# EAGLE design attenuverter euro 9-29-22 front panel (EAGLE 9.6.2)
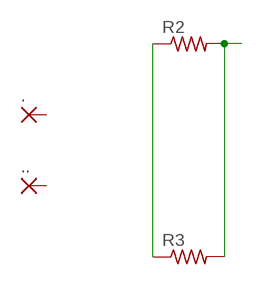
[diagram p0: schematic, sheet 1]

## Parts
.  WIREPADSMD1,27-254  [SMD1,27-2,54]
..  WIREPADSMD1,27-254  [SMD1,27-2,54]
R2  R-US_MELF0207R  [MINI_MELF-0207R]
R3  R-US_MELF0207R  [MINI_MELF-0207R]

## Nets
N$1: R2.1 R3.1
N$2: R2.2 R3.2
Unconnected: ..1(P) ...1(P)

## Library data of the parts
. .. = wirepad-NONAMES:WIREPAD: Wire PAD connect wire on PCB
R2 R3 = adafruit:R-US_: RESISTOR, American symbol

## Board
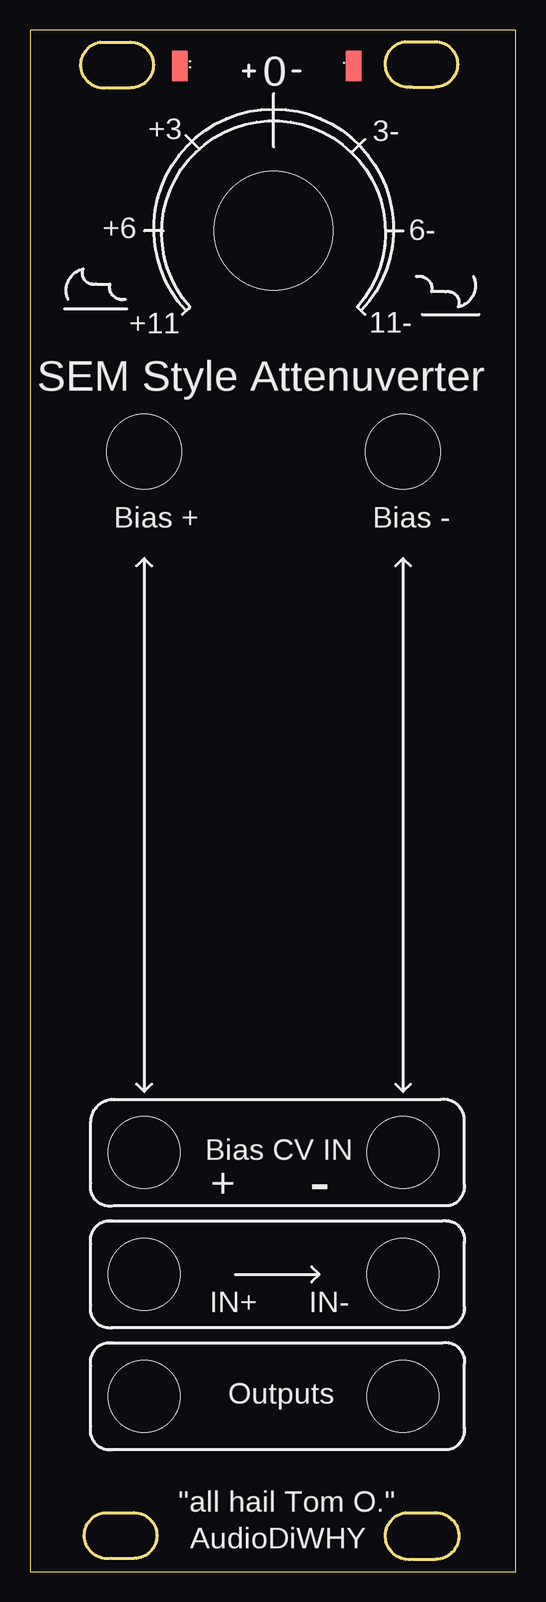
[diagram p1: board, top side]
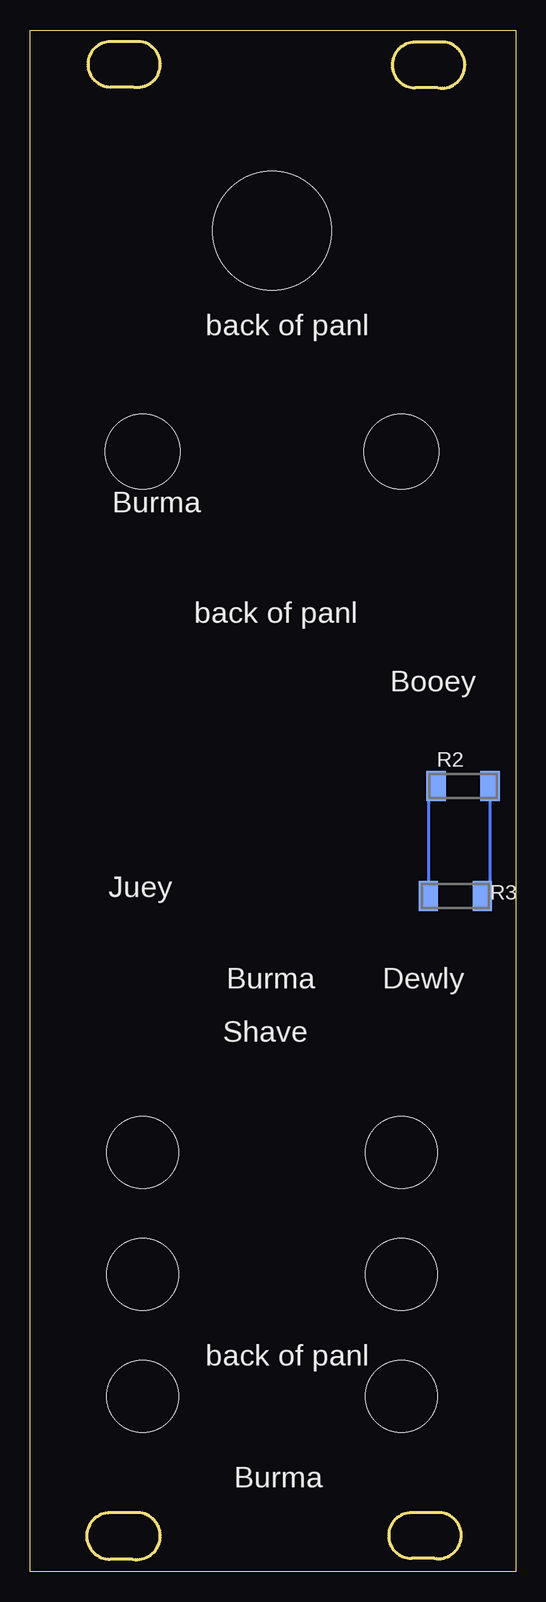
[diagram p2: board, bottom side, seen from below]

Size 40.51 x 128.5 mm. Coordinates in mm from the lower left corner, seen from the top.
Outline: 0,0 40.5,0 40.51,128.49 0,128.5 0,0
Copper layers (1*16): Top 0.035mm / dielectric 1.5mm / Bottom 0.035mm
Design rules "default": minimum track width 6mil, minimum drill 0.35mm, track to track 6mil, track to pad 6mil, pad to pad 6mil, via to via 6mil, smd to smd 6mil, copper to edge 40mil, drill to drill 6mil, minimum pad ring 10mil, minimum via ring 8mil, stop-mask expansion 4mil, vias tented up to drill 0mil, thermal gap 10mil
Holes 5.97 mm at 9.53,14.61 31.11,14.61 9.53,24.77 31.11,24.77 9.53,34.93 31.11,34.93
Holes 6.22 mm at 9.53,93.35 31.11,93.35
Holes 9.91 mm at 20.32,111.76
Milling: 16 lines

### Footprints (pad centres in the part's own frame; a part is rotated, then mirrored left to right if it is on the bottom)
SMD1,27-2,54 = smd 1.27 x 2.54: 1 0,0
MINI_MELF-0207R = smd 1.6 x 2.5: 1 -2.25,0; 2 2.25,0

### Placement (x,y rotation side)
.  27,125.5 0 top
..  12.5,125.5 0 top
R2  4.38,65.48 0 bottom
R3  5.02,56.31 0 bottom

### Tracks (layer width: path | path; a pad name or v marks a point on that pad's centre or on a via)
N$1
  Bottom 0.254: R2.1 7.27,64.85 R3.1
N$2
  Bottom 0.254: R3.2 2.13,57.01 R2.2

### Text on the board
tNames: 0 | +3 | 3- | +6 | 6- | +11 | 11- | SEM Style Attenuverter | Bias + | Bias - | Bias CV IN | + | - | IN+ | IN- | Outputs | "all hail Tom O." | AudioDiWHY
bNames: back of panl | Burma | back of panl | Booey | Juey | Dewly | Burma | Shave | back of panl | Burma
